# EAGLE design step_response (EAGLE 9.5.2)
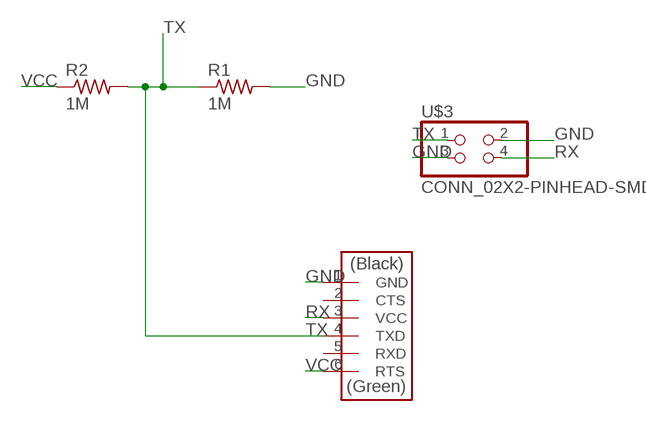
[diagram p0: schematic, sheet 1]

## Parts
R1  1M  R1206FAB  [R1206FAB]
R2  1M  R1206FAB  [R1206FAB]
U$1  CONN_06_FTDI-SMD-HEADER  [1X06SMD]
U$3  CONN_02X2-PINHEAD-SMD  [2X02SMD]

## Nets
GND: R1.2 U$1.1(GND) U$3.2 U$3.3
RX: U$1.3(VCC) U$3.4
TX: R1.1 R2.2 U$1.4(TXD) U$3.1
VCC: R2.1 U$1.6(RTS)
Unconnected: U$1.2(CTS) U$1.5(RXD)

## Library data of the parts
R1 R2 = fab:R: Resistor (US Symbol)
U$1 = fab:CONN_06_FTDI-SMD-HEADER
U$3 = fab:CONN_02X2-PINHEAD-SMD

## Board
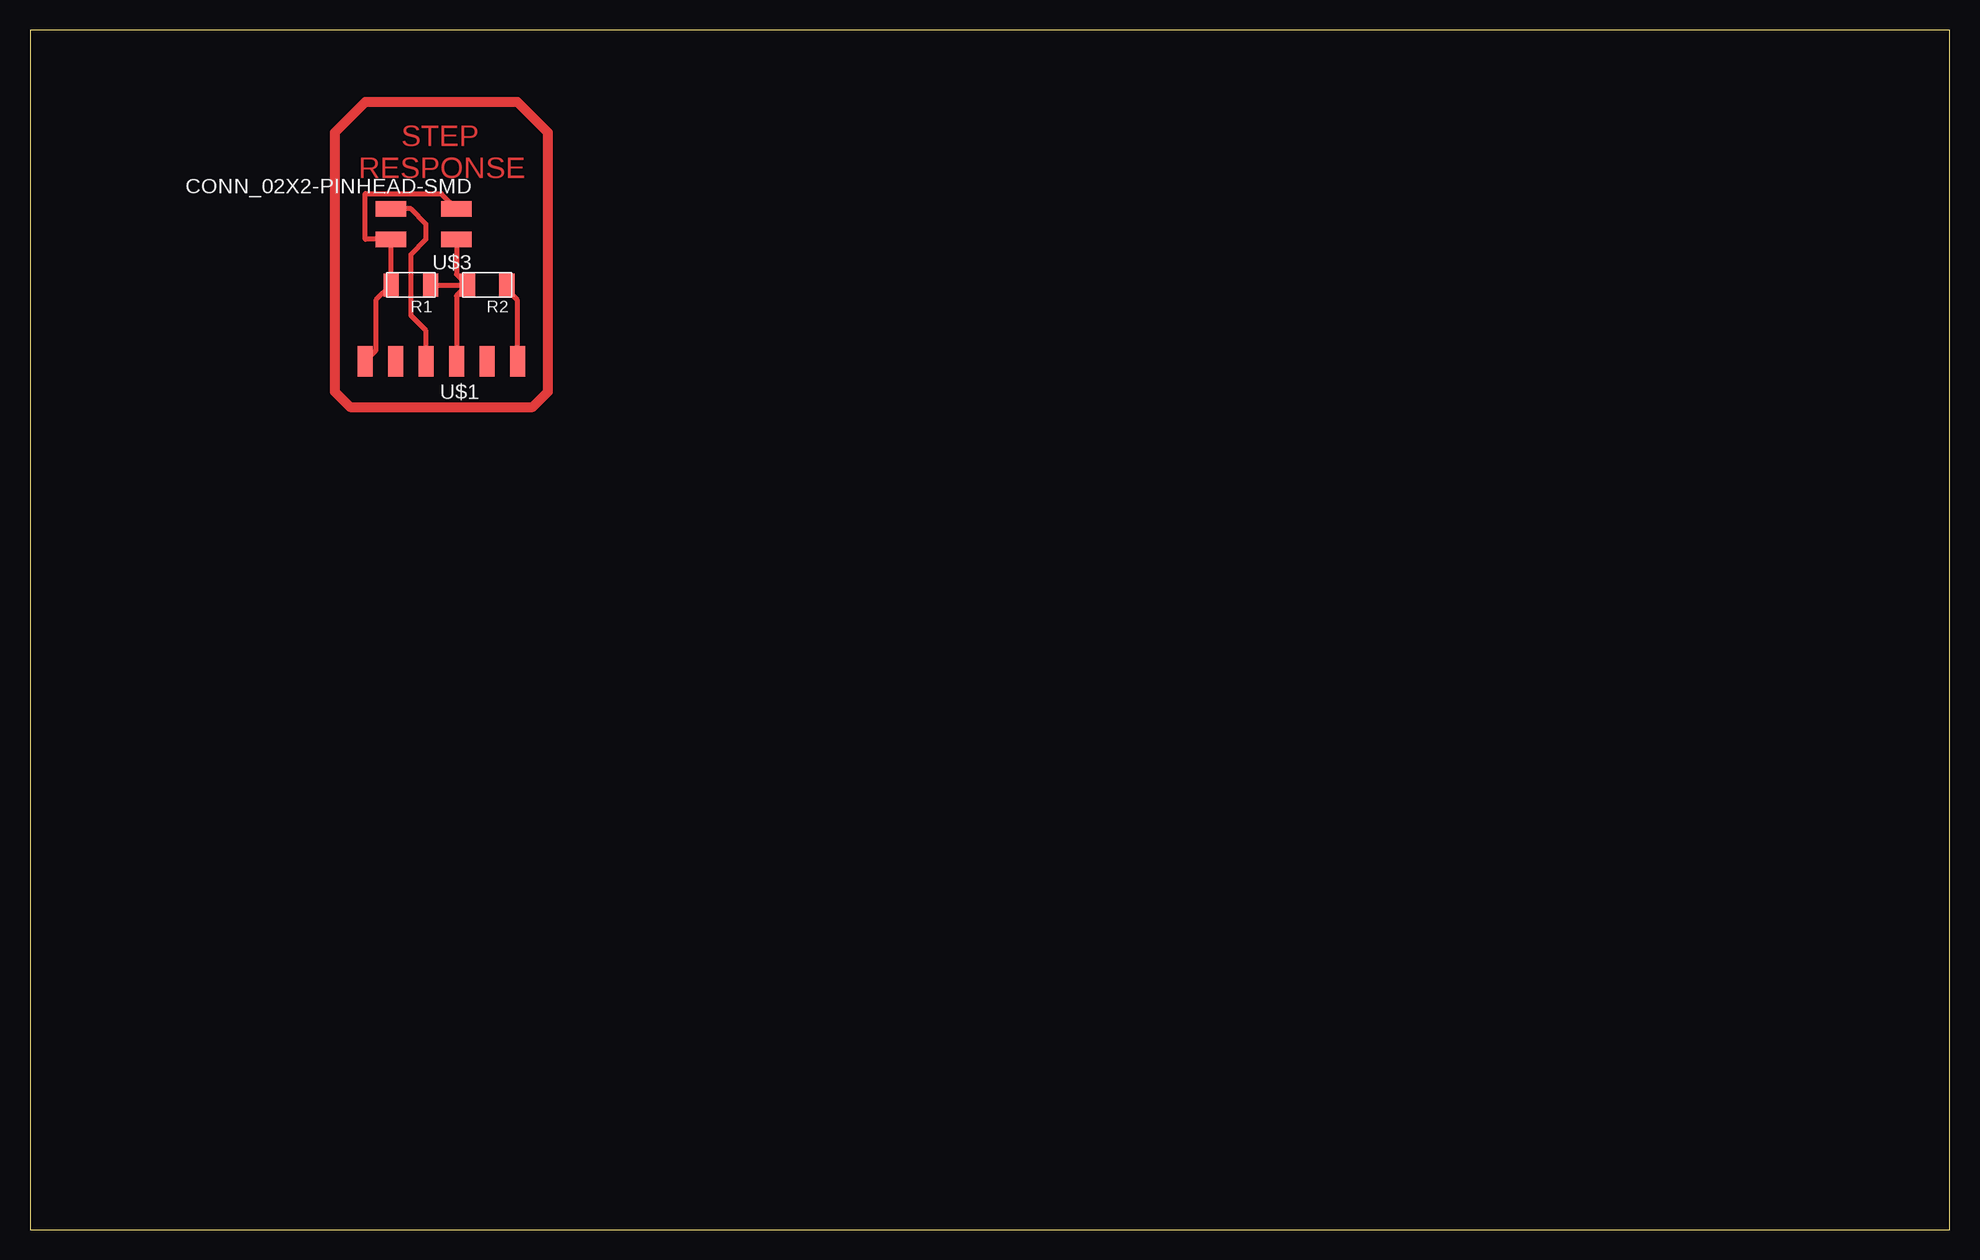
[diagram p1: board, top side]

Size 160 x 100 mm. Coordinates in mm from the lower left corner, seen from the top.
Outline: 0,0 160,0 160,100 0,100 0,0
Copper layers (1*16): Top 0.035mm / dielectric 1.5mm / Bottom 0.035mm
Design rules "default": minimum track width 6mil, minimum drill 0.35mm, track to track 6mil, track to pad 6mil, pad to pad 6mil, via to via 6mil, smd to smd 6mil, copper to edge 40mil, drill to drill 6mil, minimum pad ring 10mil, minimum via ring 8mil, stop-mask expansion 4mil, vias tented up to drill 0mil, thermal gap 10mil

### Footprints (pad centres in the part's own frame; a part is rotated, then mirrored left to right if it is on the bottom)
R1206FAB = smd 1.27 x 1.905: 1 -1.651,0; 2 1.651,0
1X06SMD = smd 2.54 x 1.27: 1 0,6.35; 2 0,3.81; 3 0,1.27; 4 0,-1.27; 5 0,-3.81; 6 0,-6.35
2X02SMD = smd 2.54 x 1.27: 1 -2.54,1.27; 2 2.92,1.27; 3 -2.54,-1.27; 4 2.92,-1.27

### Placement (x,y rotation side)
R1  31.75,78.74 180 top
R2  38.1,78.74 180 top
U$1  34.29,72.39 90 top
U$3  33.02,83.82 180 top

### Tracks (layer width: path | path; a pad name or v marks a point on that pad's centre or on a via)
GND
  Top 0.406: 35.67,85.2 U$3.3 34.29,86.36 27.94,86.36 27.94,82.55 U$3.2 R1.2 28.83,77.47 28.83,73.28 U$1.1
N$1
  Top 0.813: 25.4,91.44 25.4,69.85 26.67,68.58 41.91,68.58 43.18,69.85 43.18,91.44 40.64,93.98 27.94,93.98 25.4,91.44
RX
  Top 0.406: U$1.3 33.02,74.93 31.75,76.2 31.75,81.28 33.02,82.55 33.02,83.82 31.75,85.09 U$3.4 29.97,85.09
TX
  Top 0.406: R1.1 R2.2 | R2.2 35.56,77.85 U$1.4 | U$3.1 35.56,79.63 R2.2
VCC
  Top 0.406: U$1.6 40.64,77.47 39.75,78.36 R2.1

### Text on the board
Top: STEP / RESPONSE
